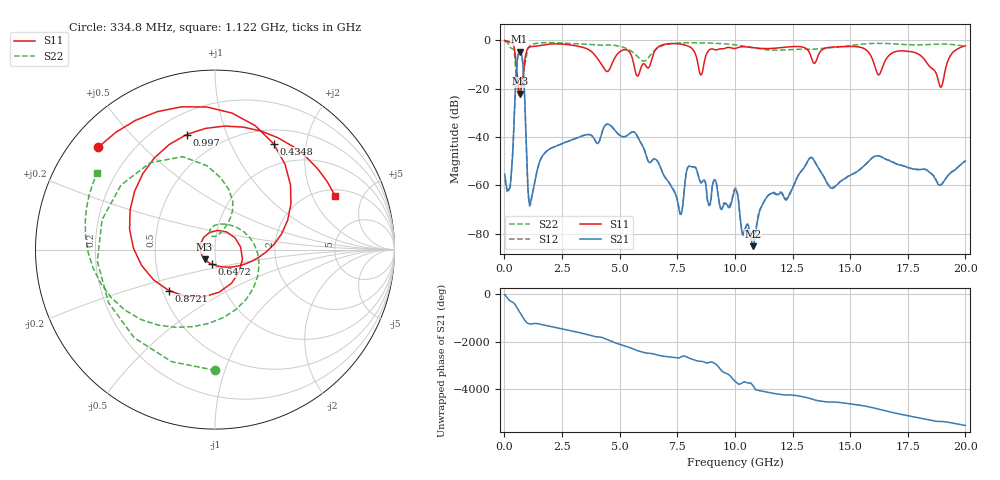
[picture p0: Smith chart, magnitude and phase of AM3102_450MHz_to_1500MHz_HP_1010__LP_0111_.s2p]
!Agilent Technologies,E8364B,MY43040894,A.07.50.67
!Agilent E8364B: A.07.50.67
!Date: Thursday, January 11, 2018 06:11:51
!Correction: S11(Full 2 Port(1,2))
!S21(Full 2 Port(1,2))
!S12(Full 2 Port(1,2))
!S22(Full 2 Port(1,2))
!S2P File: Measurements: S11, S21, S12, S22:
# Hz S  dB  R 50
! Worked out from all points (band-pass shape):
!   1601 points, 10 MHz to 20 GHz, reference 50 ohm
!   highest |S21| = -4.73 dB at 659.7 MHz (marker M1); lowest = -85.2 dB at 10.79 GHz (marker M2)
!   |S21| within 3 dB of the highest: 568.4 MHz to 779.4 MHz (211 MHz wide, 31.3 % of centre)
!   lowest |S11| = -22.1 dB at 672.2 MHz (marker M3), VSWR 1.17, Z = 44.3 - j4.78 ohm
!   |S11| at or under -10 dB: 4.217 GHz to 4.657 GHz (440.3 MHz wide, 9.92 % of centre); 16.05 GHz to 16.45 GHz (400.4 MHz wide, 2.46 % of centre); 18.38 GHz to 19.19 GHz (810.7 MHz wide, 4.32 % of centre)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
!   |S22| runs from -22.7 to -0.4 dB; largest |S21 - S12| = 0.0006
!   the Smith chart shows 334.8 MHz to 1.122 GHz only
!   S11 on the Smith chart (normalised r, x): 334.8 MHz: 0.08, +0.37; 434.8 MHz: 0.68, +1.47; 647.2 MHz: 0.95, -0.16; 872.1 MHz: 0.54, -0.28; 997 MHz: 0.32, +0.73; 1.122 GHz: 2.33, +3.01
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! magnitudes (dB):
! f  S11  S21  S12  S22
! 10 MHz  -0.1  -55.4  -57.6  -0.4
! 334.8 MHz  -1.3  -51.0  -50.7  -3.4
! 434.8 MHz  -3.4  -30.0  -30.0  -5.2
! 647.2 MHz  -21.6  -4.7  -4.8  -22.6
! 659.7 MHz  -21.9  -4.7  -4.7  -21.9
! 672.2 MHz  -22.1  -4.8  -4.8  -21.2
! 872.1 MHz  -9.3  -21.9  -21.9  -11.1
! 997 MHz  -3.6  -56.1  -56.7  -4.4
! 1.122 GHz  -2.7  -67.7  -68.4  -2.1
! 1.734 GHz  -1.8  -46.8  -46.8  -1.0
! 3.346 GHz  -2.8  -39.7  -39.7  -1.5
! 5.782 GHz  -14.8  -40.0  -40.0  -6.7
! 6.682 GHz  -2.7  -50.7  -50.6  -3.0
! 7.631 GHz  -1.5  -72.0  -71.9  -1.1
! 8.043 GHz  -2.7  -52.1  -52.0  -1.0
! 10.01 GHz  -3.4  -61.8  -61.2  -1.9
! 10.79 GHz  -3.0  -85.2  -82.7  -3.1
! 13.34 GHz  -7.8  -48.6  -48.6  -3.8
! 14.23 GHz  -2.8  -61.3  -60.9  -3.0
! 16.68 GHz  -6.3  -49.7  -49.7  -1.3
! 18.94 GHz  -19.4  -59.9  -59.7  -1.5
! 20 GHz  -2.3  -50.1  -49.8  -2.5
